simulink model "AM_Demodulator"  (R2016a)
settings: Solver=ode3  StartTime=0.0  StopTime=6  FixedStep=1/5000000  RelTol=1e-3
libraries: dsparch4 x4

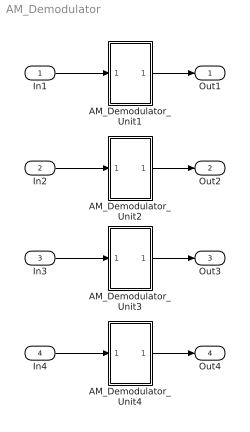
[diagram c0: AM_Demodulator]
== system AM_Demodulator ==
  In1 : Inport
  In2 : Inport  Port=2
  In3 : Inport  Port=3
  In4 : Inport  Port=4
  AM_Demodulator_Unit1 : Subsystem
  AM_Demodulator_Unit2 : Subsystem
  AM_Demodulator_Unit3 : Subsystem
  AM_Demodulator_Unit4 : Subsystem
  Out1 : Outport
  Out2 : Outport  Port=2
  Out3 : Outport  Port=3
  Out4 : Outport  Port=4
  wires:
  In1/1 -> AM_Demodulator_Unit1/1(In1)
  AM_Demodulator_Unit1/1(Out1) -> Out1/1
  In2/1 -> AM_Demodulator_Unit2/1(In1)
  AM_Demodulator_Unit2/1(Out1) -> Out2/1
  In3/1 -> AM_Demodulator_Unit3/1(In1)
  AM_Demodulator_Unit3/1(Out1) -> Out3/1
  In4/1 -> AM_Demodulator_Unit4/1(In1)
  AM_Demodulator_Unit4/1(Out1) -> Out4/1

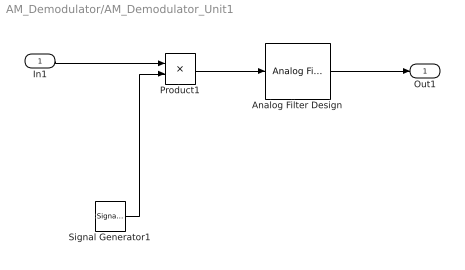
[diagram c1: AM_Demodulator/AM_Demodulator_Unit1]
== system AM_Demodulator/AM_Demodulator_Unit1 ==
  In1 : Inport
  Analog Filter Design : dsparch4/Analog Filter Design  method=Butterworth  filttype=Lowpass  N=8  Wlo=45000*2*pi  Whi=80  Rp=2  Rs=40
  Product1 : Product
  Signal Generator1 : SignalGenerator  Frequency=500000
  Out1 : Outport
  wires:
  Product1/1 -> Analog Filter Design/1
  In1/1 -> Product1/1
  Signal Generator1/1 -> Product1/2
  Analog Filter Design/1 -> Out1/1

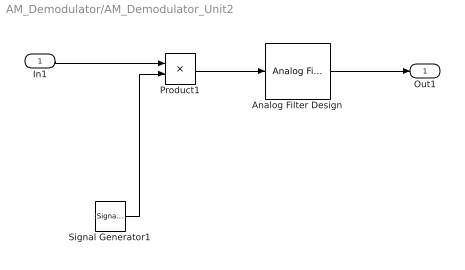
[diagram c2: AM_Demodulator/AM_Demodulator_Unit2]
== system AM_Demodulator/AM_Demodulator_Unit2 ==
  In1 : Inport
  Analog Filter Design : dsparch4/Analog Filter Design  method=Butterworth  filttype=Lowpass  N=8  Wlo=45000*2*pi  Whi=80  Rp=2  Rs=40
  Product1 : Product
  Signal Generator1 : SignalGenerator  Frequency=500000
  Out1 : Outport
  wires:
  Product1/1 -> Analog Filter Design/1
  In1/1 -> Product1/1
  Signal Generator1/1 -> Product1/2
  Analog Filter Design/1 -> Out1/1

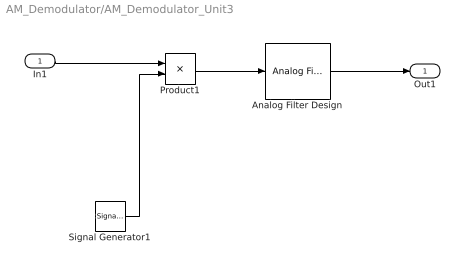
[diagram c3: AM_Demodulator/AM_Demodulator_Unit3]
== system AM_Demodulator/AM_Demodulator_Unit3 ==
  In1 : Inport
  Analog Filter Design : dsparch4/Analog Filter Design  method=Butterworth  filttype=Lowpass  N=8  Wlo=45000*2*pi  Whi=80  Rp=2  Rs=40
  Product1 : Product
  Signal Generator1 : SignalGenerator  Frequency=500000
  Out1 : Outport
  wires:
  Product1/1 -> Analog Filter Design/1
  In1/1 -> Product1/1
  Signal Generator1/1 -> Product1/2
  Analog Filter Design/1 -> Out1/1

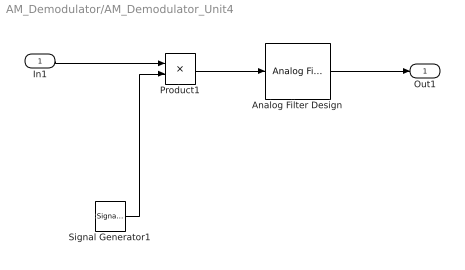
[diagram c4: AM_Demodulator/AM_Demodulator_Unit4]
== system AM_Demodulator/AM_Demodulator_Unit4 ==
  In1 : Inport
  Analog Filter Design : dsparch4/Analog Filter Design  method=Butterworth  filttype=Lowpass  N=8  Wlo=45000*2*pi  Whi=80  Rp=2  Rs=40
  Product1 : Product
  Signal Generator1 : SignalGenerator  Frequency=500000
  Out1 : Outport
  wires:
  Product1/1 -> Analog Filter Design/1
  In1/1 -> Product1/1
  Signal Generator1/1 -> Product1/2
  Analog Filter Design/1 -> Out1/1
